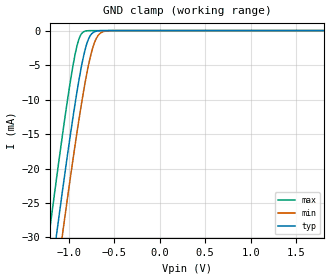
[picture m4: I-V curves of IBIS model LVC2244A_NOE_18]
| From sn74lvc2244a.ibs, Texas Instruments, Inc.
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[Model]   LVC2244A_NOE_18
Model_type  Input
Vinl=0.5775
Vinh=1.2675
| variable   typ   min   max
C_comp   5.36pF   4.98pF   5.76pF
[Temperature Range]   40   100   -40
| Ambient temperature   25   85   -40
[Voltage range]   1.8   1.65   1.95
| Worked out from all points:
|   GND clamp passes 1 mA (typ) near -0.77 V on its own axis
[GND Clamp]
| LVC2244A_NOE_18
|   Voltage   I(typ)   I(min)   I(max)
-5V       -443mA     -448.4mA   -436.3mA
-1.225V   -38.95mA   -45.29mA   -30.81mA
-1.2V     -36.43mA   -42.78mA   -28.28mA
-1.13V    -29.46mA   -35.8mA    -21.3mA
-1.07V    -23.6mA    -29.93mA   -15.5mA
-1.055V   -22.16mA   -28.48mA   -14.08mA
-955mV    -12.94mA   -19.06mA   -5.398mA
-885mV    -7.147mA   -12.88mA   -1.216mA
-780mV    -1.214mA   -4.964mA   -14.58uA
-720mV    -205uA     -1.928mA   -870.6nA
-655mV    -22.28uA   -427.1uA   -40.85nA
1.8V      5.068pA    10.93pA    4.764pA
